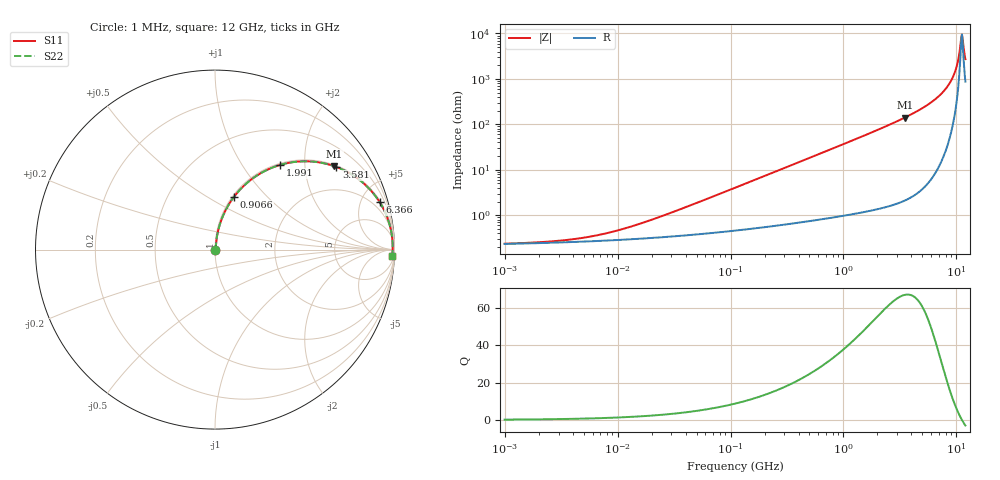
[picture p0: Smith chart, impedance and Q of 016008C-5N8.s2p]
# MHz S MA R 50
!Freq  MagS11  AngS11  MagS21  AngS21  MagS12  AngS12  MagS22  AngS22
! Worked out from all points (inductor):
!   801 points, 1 MHz to 12 GHz, reference 50 ohm
!   read as one part in series: L = 5.8 nH near 27.73 MHz
!   highest Q = 67 at 3.498 GHz (marker M1), where L = 6.43 nH
!   self-resonance near 11.05 GHz
!   S11 on the Smith chart (normalised r, x): 1 MHz: 1.00, +0.00; 906.6 MHz: 1.02, +0.67; 1.991 GHz: 1.03, +1.50; 3.581 GHz: 1.04, +2.91; 6.366 GHz: 1.16, +6.87; 12 GHz: 18, -52
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1  0.00236 8.8  0.9977 -0.0  0.9977 -0.0  0.00236 8.8
4.822396  0.003147 33.7  0.9974 -0.1  0.9974 -0.1  0.003147 33.7
9.98618  0.004609 51.7  0.9972 -0.2  0.9972 -0.2  0.004609 51.7
22.98406  0.00895 68.4  0.9967 -0.5  0.9967 -0.5  0.00895 68.4
110.8382  0.04044 81.2  0.9946 -2.3  0.9946 -2.3  0.04044 81.2
528.267  0.1882 76.9  0.9748 -10.8  0.9748 -10.8  0.1882 76.9
906.5806  0.3131 70.2  0.941 -18.2  0.941 -18.2  0.3131 70.2
1351.362  0.4432 62.4  0.8866 -26.3  0.8866 -26.3  0.4432 62.4
1990.847  0.5946 52.5  0.7934 -36.5  0.7934 -36.5  0.5946 52.5
2517.778  0.6895 45.5  0.7132 -43.6  0.7132 -43.6  0.6895 45.5
3497.75  0.8106 35.0  0.5736 -54.1  0.5736 -54.1  0.8106 35.0
3580.854  0.8184 34.2  0.5626 -54.9  0.5626 -54.9  0.8184 34.2
4916.534  0.9064 24.1  0.4079 -65.0  0.4079 -65.0  0.9064 24.1
6365.558  0.9543 16.1  0.2779 -72.6  0.2779 -72.6  0.9543 16.1
7863.54  0.9781 9.9  0.1724 -77.8  0.1724 -77.8  0.9781 9.9
9160.196  0.9873 5.6  0.09736 -79.7  0.09736 -79.7  0.9873 5.6
9944.836  0.9896 3.3  0.05753 -77.9  0.05753 -77.9  0.9896 3.3
10301.36  0.99 2.3  0.04075 -74.6  0.04075 -74.6  0.99 2.3
10796.69  0.99 1.0  0.01953 -58.6  0.01953 -58.6  0.99 1.0
11053.21  0.9898 0.3  0.01158 -27.7  0.01158 -27.7  0.9898 0.3
11449.47  0.9892 -0.7  0.01586 46.6  0.01586 46.6  0.9892 -0.7
12000  0.9878 -2.0  0.03629 69.4  0.03629 69.4  0.9878 -2.0
